FUNCTION_BLOCK Caneoseries5x_AOI
VAR_INPUT
END_VAR
VAR_OUTPUT
END_VAR
VAR
	DN_Struct : DisplayedNumber_Struct;
	String_Struct : StringToBytes;
	AC_Struct : ActiveScenes_Struct;
END_VAR

gvl.caneoSeries52_PDout_port1.activeScenesSctruct.num := gvl.caneoSeries52_PDout_port1.ActiveScenes;

gvl.ActiveScenes_byte0_port1 :=	gvl.caneoSeries52_PDout_port1.activeScenesSctruct.bytes[1];
gvl.ActiveScenes_byte1_port1 := gvl.caneoSeries52_PDout_port1.activeScenesSctruct.bytes[0];


//displayed number
gvl.caneoSeries52_PDout_port1.displayedNumberStuct.num := gvl.caneoSeries52_PDout_port1.DisplayedNumber;

gvl.Number_byte0_port1 := gvl.caneoSeries52_PDout_port1.displayedNumberStuct.bytes[3];
gvl.Number_byte1_port1 := gvl.caneoSeries52_PDout_port1.displayedNumberStuct.bytes[2];
gvl.Number_byte2_port1 := gvl.caneoSeries52_PDout_port1.displayedNumberStuct.bytes[1];
gvl.Number_byte3_port1 := gvl.caneoSeries52_PDout_port1.displayedNumberStuct.bytes[0];

gvl.caneoSeries52_PDout_port1.stringToBytes.str := gvl.caneoSeries52_PDout_port1.TextToDisplay;

gvl.String_byte0_port1 := gvl.caneoSeries52_PDout_port1.stringToBytes.bytes[0];
gvl.String_byte1_port1 := gvl.caneoSeries52_PDout_port1.stringToBytes.bytes[1];
gvl.String_byte2_port1 := gvl.caneoSeries52_PDout_port1.stringToBytes.bytes[2];
gvl.String_byte3_port1 := gvl.caneoSeries52_PDout_port1.stringToBytes.bytes[3];
gvl.String_byte4_port1 := gvl.caneoSeries52_PDout_port1.stringToBytes.bytes[4];
gvl.String_byte5_port1 := gvl.caneoSeries52_PDout_port1.stringToBytes.bytes[5];

//example usage writing to PDout
//caneoseries5x();
//gvl.caneoSeries52_PDout_port1.Mode := 1;
//gvl.caneoSeries52_PDout_port1.TextColor := 1;
//gvl.caneoSeries52_PDout_port1.DisplayedNumber := 12345;
//gvl.caneoSeries52_PDout_port1.TextSelect := 1;
//gvl.caneoSeries52_PDout_port1.ActiveScenes := 1;

END_FUNCTION_BLOCK
